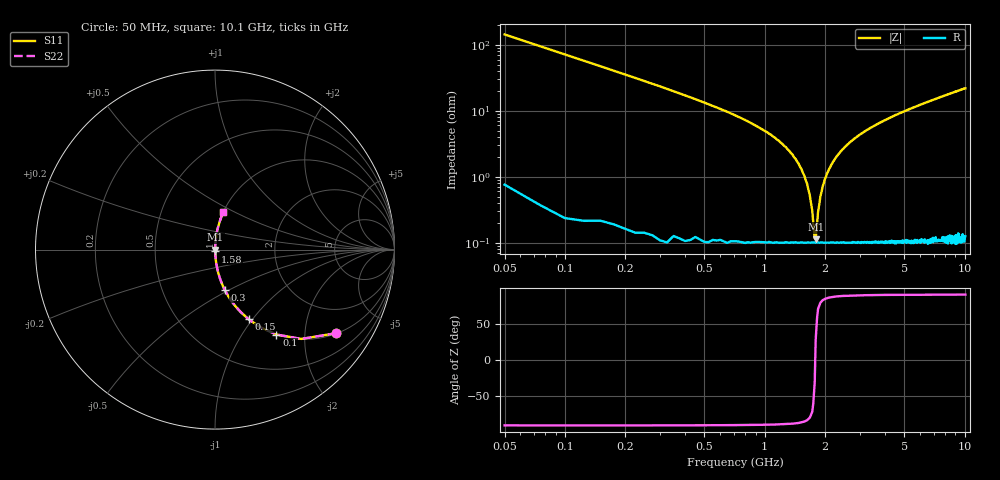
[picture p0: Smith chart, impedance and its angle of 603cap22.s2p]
! AVX Thin Film Operation		Date: November 2004
! Description: Accu-P® Series, Thin Film, SMD, RF Capacitor
! Part Number: 06033J220FBT
! 50 MHz  -  10.05 GHz
! Serial Measurements
# hz S db R 50
!	S11		S21		S12		S22
!	dB	Phase	dB	Phase	dB	Phase	dB	Phase
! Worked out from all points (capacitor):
!   400 points, 50 MHz to 10.1 GHz, reference 50 ohm
!   read as one part in series: C = 22 pF near 100 MHz
!   lowest |Z| = 113 mohm at 1.8 GHz (marker M1)
!   series resonance near 1.791 GHz, so ESL is about 360 pH
!   S11 on the Smith chart (normalised r, x): 50 MHz: 1.01, -2.89; 100 MHz: 1.00, -1.44; 150 MHz: 1.00, -0.96; 300 MHz: 1.00, -0.47; 1.58 GHz: 1.00, -0.02; 10.1 GHz: 1.00, +0.44
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5e7  -1.72 -34.6  -4.92 55.1  -4.92 55.1  -1.72 -34.6
1e8  -4.67 -54.1  -1.83 35.7  -1.83 35.7  -4.67 -54.1
1.5e8  -7.30 -64.2  -0.91 25.5  -0.91 25.5  -7.30 -64.2
3e8  -12.80 -76.5  -0.24 13.2  -0.24 13.2  -12.80 -76.5
6e8  -19.50 -83.3  -0.06 6.1  -0.06 6.1  -19.50 -83.3
1.28e9  -31.10 -86.3  -0.01 1.6  -0.01 1.6  -31.10 -86.3
1.58e9  -39.70 -83.9  -0.01 0.6  -0.01 0.6  -39.70 -83.9
1.68e9  -45.40 -79.0  -0.01 0.3  -0.01 0.3  -45.40 -79.0
1.73e9  -50.20 -70.9  -0.01 0.2  -0.01 0.2  -50.20 -70.9
1.78e9  -58.60 -31.2  -0.01 0.0  -0.01 0.0  -58.60 -31.2
1.8e9  -59.00 27.6  -0.01 -0.0  -0.01 -0.0  -59.00 27.6
1.85e9  -50.70 69.8  -0.01 -0.2  -0.01 -0.2  -50.70 69.8
1.9e9  -46.00 78.2  -0.01 -0.3  -0.01 -0.3  -46.00 78.2
1.95e9  -43.00 81.5  -0.01 -0.4  -0.01 -0.4  -43.00 81.5
2.05e9  -39.10 84.2  -0.01 -0.6  -0.01 -0.6  -39.10 84.2
2.2e9  -35.40 85.6  -0.01 -1.0  -0.01 -1.0  -35.40 85.6
2.65e9  -29.70 86.4  -0.01 -1.9  -0.01 -1.9  -29.70 86.4
3.4e9  -25.10 85.8  -0.02 -3.2  -0.02 -3.2  -25.10 85.8
5.08e9  -20.00 83.7  -0.05 -5.7  -0.05 -5.7  -20.00 83.7
6.75e9  -17.10 81.5  -0.10 -8.1  -0.10 -8.1  -17.10 81.5
8.43e9  -15.00 79.3  -0.15 -10.3  -0.15 -10.3  -15.00 79.3
1.01e10  -13.40 77.3  -0.21 -12.4  -0.21 -12.4  -13.40 77.3
